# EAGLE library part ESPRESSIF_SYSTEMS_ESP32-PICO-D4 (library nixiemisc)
ESP32 BLUETOOTH MODULE
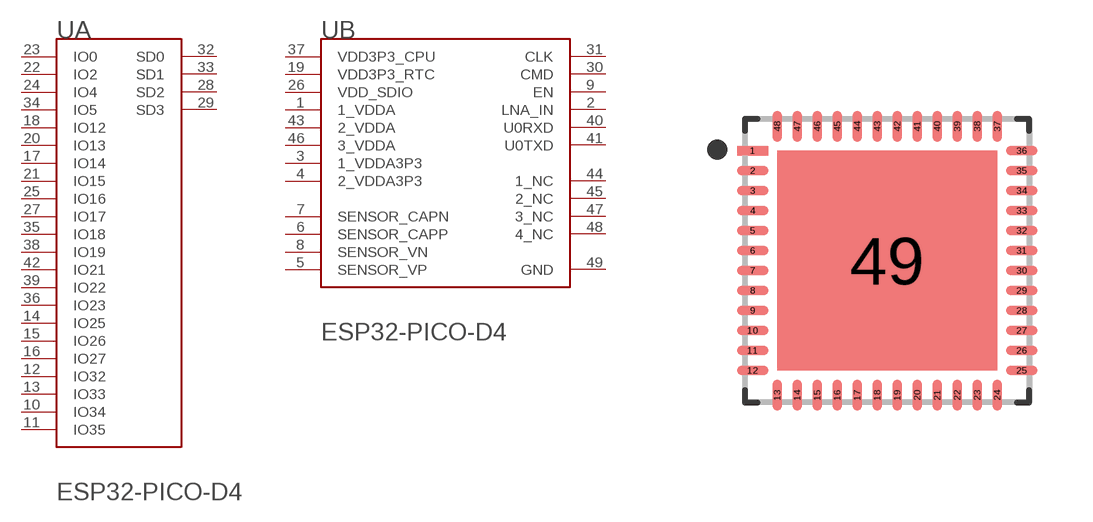
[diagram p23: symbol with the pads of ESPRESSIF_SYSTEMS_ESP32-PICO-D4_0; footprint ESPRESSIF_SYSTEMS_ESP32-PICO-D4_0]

Designator prefix U; gates A=ESPRESSIF_SYSTEMS_ESP32-PICO-D4_0_0 B=ESPRESSIF_SYSTEMS_ESP32-PICO-D4_0_1

## ESPRESSIF_SYSTEMS_ESP32-PICO-D4ESPRESSIF_SYSTEMS_ESP32-PICO-D4_0_0 (CENTROID_NOT_SPECIFIED: No; DATASHEET: https://www.espressif.com/sites/default/files/documentation/esp32-pico-d4_datasheet_en.pdf; DATA_RATE: 150mbps; DEVICE_CLASS_L1: Integrated Circuits (ICs); DEVICE_CLASS_L2: RF Semiconductors and Devices; DEVICE_CLASS_L3: Transceivers; DIGIKEY_DESCRIPTION: IC ESP32 WIFI BLUETOOTH; DIGIKEY_PART_NUMBER: 1904-1029-1-ND; FOOTPRINT_PARAMETERS_0: {"fp_type":"QFN","params":{"N1":{"nom":12,"long name":"Leads on long side","min":null,"max":null,"short name":"N1","type":"count"},"N2":{"nom":12,"long name":"Leads on wide side","min":null,"max":null,"short name":"N2","type":"count"},"A":{"nom":940000,"long name":"Height","min":840000,"max":1040000,"short name":"A","type":"measurement"},"A1":{"nom":false,"long name":"Package clearance","min":0,"max":50000,"short name":"A1","type":"measurement"},"A2":{"nom":false,"long name":"Package height","min":800000,"max":false,"short name":"A2","type":"measurement"},"D":{"nom":7000000,"long name":"Package length","min":6900000,"max":7100000,"short name":"D","type":"measurement"},"E":{"nom":7000000,"long name":"Package width","min":6900000,"max":7100000,"short name":"E","type":"measurement"},"B":{"nom":250000,"long name":"Lead width","min":200000,"max":300000,"short name":"B","type":"measurement"},"C":{"nom":260000,"long name":"Lead thickness","min":null,"max":null,"short name":"C","type":"measurement"},"L":{"nom":400000,"long name":"Lead foot length","min":325000,"max":475000,"short name":"L","type":"measurement"},"e":{"nom":500000,"long name":"Lead pitch","min":null,"max":null,"short name":"e","type":"measurement"},"HT":{"default":"Yes","long name":"Thermal pad","type":"multichoiceparent","short name":"HT","children":["D2","E2","PC"]},"offset x":{"nom":0,"long name":"X Center offset","min":null,"max":null,"short name":"offset x","type":"measurement"},"offset y":{"nom":0,"long name":"Y Center offset","min":null,"max":null,"short name":"offset y","type":"measurement"},"LS":{"default":"Rounded rectangle","long name":"Land shape","type":"multichoice","short name":"LS"},"LS1":{"default":"Rectangle","long name":"Land shape (Pin 1)","type":"multichoice","short name":"LS1"},"solder toe":{"nom":200000,"long name":"Solder fillet (toe)","min":null,"max":null,"short name":"solder toe","type":"fixedmeasurement"},"solder heel":{"nom":0,"long name":"Solder fillet (heel)","min":null,"max":null,"short name":"solder heel","type":"fixedmeasurement"},"solder side":{"nom":-40000,"long name":"Solder fillet (side)","min":null,"max":null,"short name":"solder side","type":"fixedmeasurement"},"courtyard":{"nom":100000,"long name":"Courtyard","min":null,"max":null,"short name":"courtyard","type":"fixedmeasurement"},"SF":{"default":"C","long name":"Packing level","type":"multichoiceparent","short name":"SF","help":"http://support.upverter.com/customer/portal/articles/978783-what-is-a-footprint-packing-level","children":["solder toe","solder heel","solder side","courtyard"]},"D2":{"nom":5400000,"long name":"Thermal pad length","min":5300000,"max":5500000,"short name":"D2","type":"measurement"},"E2":{"nom":5400000,"long name":"Thermal pad width","min":5300000,"max":5500000,"short name":"E2","type":"measurement"},"PC":{"long name":"Paste coverage (%)","type":"percentage","short name":"PC","value":40}}}; HEIGHT: 1.040mm; INTERFACE: I2C,SPI,UART,I2S,Other; IPC_LAND_PATTERN_NAME: QFN50P700X700X94-48; LEAD_FREE: yes; MAX_FREQUENCY: 2484MHz; MAX_SUPPLY_VOLTAGE: 3.6V; MF: Espressif Systems; MFG_PACKAGE_IDENT: ESP32-PICO-D4; MFG_PACKAGE_IDENT_DATE: 0; MFG_PACKAGE_IDENT_REV: 0; MIN_SUPPLY_VOLTAGE: 2.7V; MOUSER_PART_NUMBER: 356-ESP32-PICO-D4; MPN: ESP32-PICO-D4; NOMINAL_SUPPLY_CURRENT: 80mA; NUMBER_OF_ADC_CHANNELS: 18; NUMBER_OF_GPIO: 22; PACKAGE: QFN48; PREFIX: U; ROHS: yes; SENSITIVITY: -97dBm; TEMPERATURE_RANGE_HIGH: +85°C; TEMPERATURE_RANGE_LOW: -40°C; VERIFICATION_VERSION: 0.0.0.1)  [ESPRESSIF_SYSTEMS_ESP32-PICO-D4_0]
1  B:1_VDDA  pwr
2  B:LNA_IN
3  B:1_VDDA3P3  pwr
4  B:2_VDDA3P3  pwr
5  B:SENSOR_VP  in
6  B:SENSOR_CAPP  in
7  B:SENSOR_CAPN  in
8  B:SENSOR_VN  in
9  B:EN  in
10  A:IO34  in
11  A:IO35  in
12  A:IO32
13  A:IO33
14  A:IO25
15  A:IO26
16  A:IO27
17  A:IO14
18  A:IO12
19  B:VDD3P3_RTC  pwr
20  A:IO13
21  A:IO15
22  A:IO2
23  A:IO0
24  A:IO4
25  A:IO16
26  B:VDD_SDIO  pwr
27  A:IO17
28  A:SD2
29  A:SD3
30  B:CMD
31  B:CLK  in
32  A:SD0
33  A:SD1
34  A:IO5
35  A:IO18
36  A:IO23
37  B:VDD3P3_CPU  pwr
38  A:IO19
39  A:IO22
40  B:U0RXD  in
41  B:U0TXD  out
42  A:IO21
43  B:2_VDDA  pwr
44  B:1_NC  pas
45  B:2_NC  pas
46  B:3_VDDA  pwr
47  B:3_NC  pas
48  B:4_NC  pas
49  B:GND  pwr

## Footprint ESPRESSIF_SYSTEMS_ESP32-PICO-D4_0 (pad centres in mm)
ESP32 BLUETOOTH MODULE
smd 0.785 x 0.242: 1 -3.363,2.75; 2 -3.363,2.25; 3 -3.363,1.75; 4 -3.363,1.25; 5 -3.363,0.75; 6 -3.363,0.25; 7 -3.363,-0.25; 8 -3.363,-0.75; 9 -3.363,-1.25; 10 -3.363,-1.75; 11 -3.363,-2.25; 12 -3.363,-2.75; 25 3.363,-2.75; 26 3.363,-2.25; 27 3.363,-1.75; 28 3.363,-1.25; 29 3.363,-0.75; 30 3.363,-0.25; 31 3.363,0.25; 32 3.363,0.75; 33 3.363,1.25; 34 3.363,1.75; 35 3.363,2.25; 36 3.363,2.75
smd 0.242 x 0.785: 13 -2.75,-3.363; 14 -2.25,-3.363; 15 -1.75,-3.363; 16 -1.25,-3.363; 17 -0.75,-3.363; 18 -0.25,-3.363; 19 0.25,-3.363; 20 0.75,-3.363; 21 1.25,-3.363; 22 1.75,-3.363; 23 2.25,-3.363; 24 2.75,-3.363; 37 2.75,3.363; 38 2.25,3.363; 39 1.75,3.363; 40 1.25,3.363; 41 0.75,3.363; 42 0.25,3.363; 43 -0.25,3.363; 44 -0.75,3.363; 45 -1.25,3.363; 46 -1.75,3.363; 47 -2.25,3.363; 48 -2.75,3.363
smd 5.5 x 5.5: 49 0,0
